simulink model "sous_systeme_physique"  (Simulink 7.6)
settings: Solver=ode15s  StartTime=0.0  StopTime=1  RelTol=1e-3
StopFcn:
  | close all
  | 
  | load vitesse_position2.mat
  | plot(x(1,:),x(2,:),x(1,:),x(3,:))
  | axis([0 1 0 125])
  | grid
  | gtext('position (rad)')
  | gtext('vitesse (rad/s)')
  | title('Position et vitesse angulaires')
  | 
  | delete *.mat
undefined symbols (not defined in the file or in its folder): sigbuilder_block
libraries: fl_lib x6, nesl_utility x4, elec_lib x1

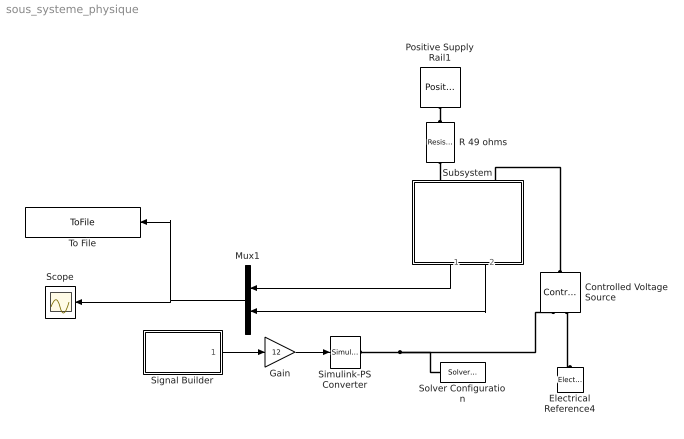
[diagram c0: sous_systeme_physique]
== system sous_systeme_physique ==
  Controlled Voltage Source : fl_lib/Electrical/Electrical Sources/Controlled Voltage Source  DialogController=NetworkEngine.DynNeDlgSource  SystemSampleTime=-1  i_Log=off  v_Log=off  LocalVarNames=|i|v  LocalVarDescs=|i|v  LocalVarLogging=[0 0]
  Electrical Reference4 : fl_lib/Electrical/Electrical Elements/Electrical Reference  DialogController=NetworkEngine.DynNeDlgSource  SystemSampleTime=-1  i_Log=off  LocalVarNames=|i  LocalVarDescs=|i  LocalVarLogging=[]
  Gain : Gain  Gain=12
  Mux1 : Mux  Inputs=2
  Positive Supply Rail1 : elec_lib/Sources/Positive Supply Rail  DialogController=NetworkEngine.DynNeDlgSource  SystemSampleTime=-1  v0=12 V  current_Log=off  voltage_Log=off  power_Log=off  LocalVarNames=|current|voltage|power  LocalVarDescs=|Current (A)|Voltage (V)|Power (W)  LocalVarLogging=[0 0 0]
  R 49 ohms : fl_lib/Electrical/Electrical Elements/Resistor  DialogController=NetworkEngine.DynNeDlgSource  SystemSampleTime=-1  R=49 Ohm  i_Log=off  v_Log=off  LocalVarNames=|i|v  LocalVarDescs=|i|v  LocalVarLogging=[0 0]
  Scope : Scope
  Signal Builder : Subsystem  Tag=STV Subsys  LoadFcn=sigbuilder_block('load');  StartFcn=sigbuilder_block('start');  StopFcn=sigbuilder_block('stop');  ClipboardFcn=sigbuilder_block('clipboard');
  Simulink-PS Converter : nesl_utility/Simulink-PS Converter  DialogController=NetworkEngine.DynNeUtilDlgSource  SystemSampleTime=-1  PhysicalDomain=network_engine_domain  LeftPortType=input  RightPortType=output  SubClassName=ps_input  Unit=1  AffineConversion=off  InputFilterTimeConstant=.001  UdotUserProvided=0
  Solver Configuration : nesl_utility/Solver Configuration  DialogController=NetworkEngine.DynNeUtilDlgSource  SystemSampleTime=-1  PhysicalDomain=network_engine_domain  LeftPortType=input  RightPortType=generic  SubClassName=solver  Accelerate=off  Profile=off  ResidualTolerance=1e-9  MaxNonlinIter=12  MaxModeIter=2  DoFixedCost=off  UseLocalSampling=off  DoDC=off  LinearAlgebra=Sparse  LocalSolverSampleTime=.001  LocalSolverChoice=NE_BACKWARD_EULER_ADVANCER  UseLocalSolver=off
  Subsystem : Subsystem
  To File : ToFile  Filename=vitesse_position2  MatrixName=x
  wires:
  Gain/1 -> Simulink-PS Converter/1
  Signal Builder/1(Signal 2) -> Gain/1
  Subsystem/1(W) -> Mux1/1
  Mux1/1 -> Scope/1, To File/1
  Subsystem/2(A) -> Mux1/2
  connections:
  Positive Supply Rail1/RConn1 -- R 49 ohms/LConn1
  R 49 ohms/RConn1 -- Subsystem/LConn1
  Controlled Voltage Source/RConn2 -- Electrical Reference4/LConn1
  Simulink-PS Converter/RConn1 -- Controlled Voltage Source/RConn1 -- Solver Configuration/RConn1
  Controlled Voltage Source/LConn1 -- Subsystem/LConn2

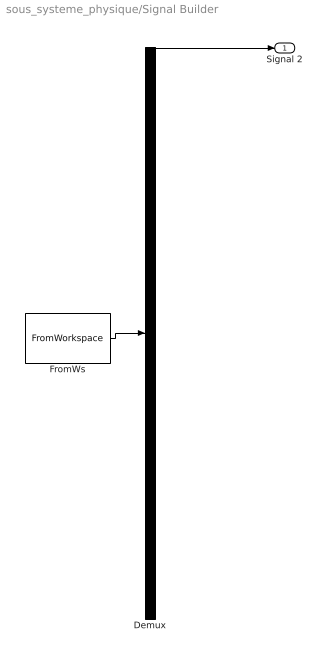
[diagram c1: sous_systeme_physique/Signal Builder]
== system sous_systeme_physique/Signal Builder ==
  Demux : Demux  Tag=STV Demux  Outputs=1
  FromWs : FromWorkspace  Tag=STV FromWs  VariableName=tuvar  SampleTime=0  SigBuilderData=DataTag0  VnvData=DataTag1
  Signal 2 : Outport  Tag=STV Outport
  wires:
  Demux/1 -> Signal 2/1
  FromWs/1 -> Demux/1

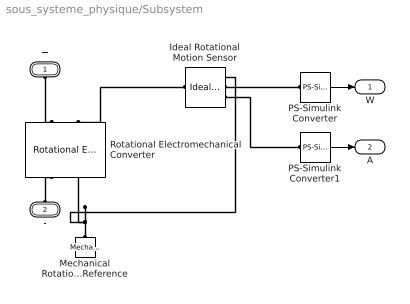
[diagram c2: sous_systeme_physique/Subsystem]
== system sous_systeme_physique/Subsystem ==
  Ideal Rotational Motion Sensor : fl_lib/Mechanical/Mechanical Sensors/Ideal Rotational Motion Sensor  DialogController=NetworkEngine.DynNeDlgSource  SystemSampleTime=-1  offset=0 rad  w_Log=off  t_Log=off  phi_Log=off  LocalVarNames=|w|t|phi  LocalVarDescs=|w|t|phi  LocalVarLogging=[0 0 0]
  Mechanical Rotational Reference : fl_lib/Mechanical/Rotational Elements/Mechanical Rotational Reference  DialogController=NetworkEngine.DynNeDlgSource  SystemSampleTime=-1  t_Log=off  LocalVarNames=|t  LocalVarDescs=|t  LocalVarLogging=0
  PS-Simulink Converter : nesl_utility/PS-Simulink Converter  DialogController=NetworkEngine.DynNeUtilDlgSource  SystemSampleTime=-1  PhysicalDomain=network_engine_domain  LeftPortType=input  RightPortType=output  SubClassName=ps_output  Unit=1  AffineConversion=off
  PS-Simulink Converter1 : nesl_utility/PS-Simulink Converter  DialogController=NetworkEngine.DynNeUtilDlgSource  SystemSampleTime=-1  PhysicalDomain=network_engine_domain  LeftPortType=input  RightPortType=output  SubClassName=ps_output  Unit=1  AffineConversion=off
  Rotational Electromechanical Converter : fl_lib/Electrical/Electrical Elements/Rotational Electromechanical Converter  DialogController=NetworkEngine.DynNeDlgSource  SystemSampleTime=-1  K=0.1 V/(rad/s)  i_Log=off  v_Log=off  t_Log=off  w_Log=off  LocalVarNames=|i|v|t|w  LocalVarDescs=|i|v|t|w  LocalVarLogging=[0 0 0 0]
  + : PMIOPort  Port=1  Side=Left
  - : PMIOPort  Port=2  Side=Left
  W : Outport
  A : Outport  Port=2
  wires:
  PS-Simulink Converter1/1 -> A/1
  PS-Simulink Converter/1 -> W/1
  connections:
  -/RConn1 -- Rotational Electromechanical Converter/RConn1
  +/RConn1 -- Rotational Electromechanical Converter/LConn1
  Ideal Rotational Motion Sensor/RConn3 -- PS-Simulink Converter1/LConn1
  Ideal Rotational Motion Sensor/RConn2 -- PS-Simulink Converter/LConn1
  Mechanical Rotational Reference/LConn1 -- Ideal Rotational Motion Sensor/RConn1 -- Rotational Electromechanical Converter/RConn2
  Ideal Rotational Motion Sensor/LConn1 -- Rotational Electromechanical Converter/LConn2
